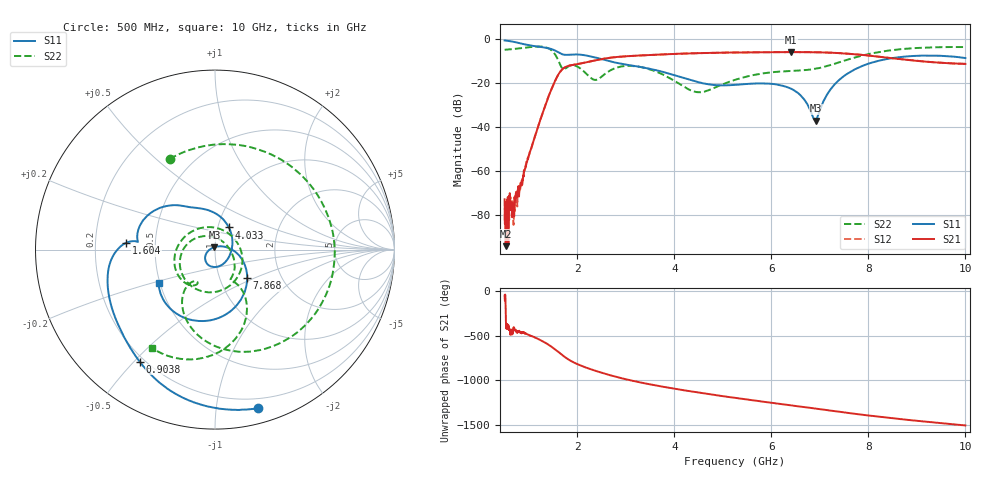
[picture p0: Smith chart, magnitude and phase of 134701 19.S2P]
!  2-Port S-parameters saved by WinCal
! VAR MeasName=S-Parameters (CALIBRATED_DATA) read from VNA (N5242A)
! VAR MeasDate=2013-7-3 16:31:10
! VAR NAME=134701 19
! VAR FILENAME=134701 19.S2P
! VAR DATE=2013-7-3 16:31:10
! VAR PHYS_PORTS=1,2
# Hz S MA R 50
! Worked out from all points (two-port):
!   1601 points, 500 MHz to 10 GHz, reference 50 ohm
!   highest |S21| = -6.04 dB at 6.402 GHz (marker M1); lowest = -94.1 dB at 523.8 MHz (marker M2)
!   |S21| within 3 dB of the highest: 2.545 GHz to 8.579 GHz (6.034 GHz wide, 108 % of centre)
!   lowest |S11| = -37.1 dB at 6.912 GHz (marker M3), VSWR 1.03, Z = 49.7 + j1.36 ohm
!   |S11| at or under -10 dB: 2.632 GHz to 8.211 GHz (5.578 GHz wide, 103 % of centre)
!   |S22| runs from -24.3 to -3.5 dB; largest |S21 - S12| = 0.0029
!   S11 on the Smith chart (normalised r, x): 500 MHz: 0.12, -1.30; 903.8 MHz: 0.18, -0.52; 1.604 GHz: 0.34, +0.03; 4.033 GHz: 1.13, +0.28; 7.868 GHz: 1.35, -0.46; 10 GHz: 0.49, -0.21
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5e8  0.9165 -74.8  0.0002285 -54.8  7.517e-05 -67.1  0.5646 116.6
5.2375e8  0.91 -78.0  1.977e-05 95.8  0.0001427 -44.2  0.5666 113.2
6.721875e8  0.8593 -97.8  0.0001539 -109.8  0.0001574 -79.7  0.5843 91.3
9.0375e8  0.7519 -123.9  0.0009812 -111.5  0.001068 -111.0  0.6243 51.6
1.165e9  0.6701 -146.7  0.008398 -171.1  0.008258 -171.4  0.6678 -4.1
1.372812e9  0.6198 -164.9  0.03939 128.3  0.03938 128.2  0.6276 -59.0
1.604375e9  0.4954 175.6  0.1525 39.1  0.152 39.0  0.3268 -123.9
1.770625e9  0.4317 174.2  0.2336 -31.4  0.233 -31.5  0.2187 -117.6
2.085312e9  0.4338 158.5  0.2782 -119.0  0.2774 -119.0  0.2026 171.1
2.37625e9  0.3755 140.7  0.3254 -174.6  0.3248 -174.6  0.1167 57.5
2.928438e9  0.2678 118.8  0.3959 100.7  0.3952 100.6  0.2374 -92.1
3.670625e9  0.1882 82.1  0.4378 17.1  0.4371 17.2  0.1718 176.8
4.032812e9  0.1456 58.0  0.4549 -17.0  0.4547 -17.0  0.1063 136.4
4.543438e9  0.1005 16.0  0.4737 -61.0  0.4739 -61.0  0.06139 50.2
5.25e9  0.09005 -51.3  0.4884 -116.6  0.4891 -116.7  0.1171 -26.1
6.401875e9  0.07397 -138.5  0.4989 160.4  0.4987 160.2  0.186 -62.2
6.835312e9  0.01951 156.2  0.4963 129.4  0.4961 129.4  0.203 -60.7
6.9125e9  0.01395 101.9  0.4946 123.9  0.4947 123.8  0.2095 -59.5
7.286562e9  0.08756 2.3  0.4808 96.8  0.4807 96.7  0.2672 -56.3
7.868438e9  0.2405 -41.8  0.4308 55.7  0.4313 55.5  0.4149 -65.4
8.420625e9  0.3535 -75.8  0.3696 20.3  0.37 20.0  0.5412 -82.2
1e10  0.3656 -149.4  0.2697 -64.4  0.2691 -64.8  0.6494 -122.8
